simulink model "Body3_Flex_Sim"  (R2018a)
settings: Solver=ode3  StartTime=0.0  StopTime=200  FixedStep=Ts  RelTol=1e-3  EnableMultiTasking=on
InitFcn:
  | run
StopFcn:
  | pl
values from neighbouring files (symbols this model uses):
  d2r = pi/180    (= 0.0174532925199)    [orbitic.m]    (also in Quan.m; run.m; runf.m)
  Int_IC = [qti', 0 0, h0i(1:3)', 0 0, wr0, Vec0'*M0, Pec0']    [run.m]
  Kq1 = I22*ww^2 - 3*wo2*(I11-I33)    [run.m]
  Kq2 = 2*I22*zet*ww    [run.m]
  Kqi = 0.0005    [run.m]
  Kr1 = (0.1*I11*I33*zet^2/Hy0) - sqrt( ((0.01^zet^4*I11^2*I33^2)/Hy0^2)+(4*I11*I33*zet^2) )    [run.m]
  Kr2 = 0.05*Kr1    [run.m]
  Kr3 = 0.04*zet*(Kr2-Hy0) * sqrt(abs(Hy0/(I11*I33)))    [run.m]
  nt = 7    [run.m]    (also in runf.m)
  r2d = 180/pi    (= 57.2957795131)    [pl.m]    (also in pl2.m; run.m; plf.m; runf.m)
  Ts = 0.001    [run.m]    (also in runf.m = 0.0005)
  wo = 0.00113    [run.m]
undefined symbols (not defined in the file or in its folder): Aflx, Bflx, Cflx, den, Dflx, DiscIntNeverNeededParam, Mode_Switch, num, Phase_Plane, RW_Steering, Vehi_3B3W
libraries: simulink x4

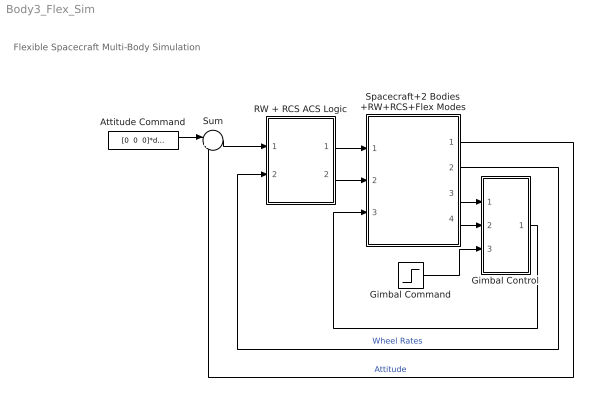
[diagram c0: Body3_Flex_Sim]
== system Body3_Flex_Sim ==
  note: Flexible Spacecraft Multi-Body Simulation
  Attitude Command : Constant  Value="[0  0  0]*d2r"
  Gimbal Control : Subsystem
  Gimbal Command : Step  After=[5, 5]*d2r  SampleTime=0
  RW + RCS ACS Logic : Subsystem
  Spacecraft+2 Bodies +RW+RCS+Flex Modes : Subsystem
  Sum : Sum  Inputs=|+-
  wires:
  Spacecraft+2 Bodies +RW+RCS+Flex Modes/2(Wrw) -> RW + RCS ACS Logic/2(wr(i))  "Wheel Rates"
  Attitude Command/1 -> Sum/1
  Spacecraft+2 Bodies +RW+RCS+Flex Modes/1(atti) -> Sum/2  "Attitude"
  Sum/1 -> RW + RCS ACS Logic/1(atter)
  RW + RCS ACS Logic/2(Trwi) -> Spacecraft+2 Bodies +RW+RCS+Flex Modes/2(Trw)
  RW + RCS ACS Logic/1(Frcs) -> Spacecraft+2 Bodies +RW+RCS+Flex Modes/1(Fjets)
  Spacecraft+2 Bodies +RW+RCS+Flex Modes/4(Gmb-dot) -> Gimbal Control/2(Grat)
  Spacecraft+2 Bodies +RW+RCS+Flex Modes/3(gimb) -> Gimbal Control/1(Gimb)
  Gimbal Control/1(Trq) -> Spacecraft+2 Bodies +RW+RCS+Flex Modes/3(Tgimb)
  Gimbal Command/1 -> Gimbal Control/3(Cmd)

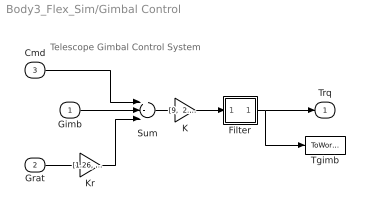
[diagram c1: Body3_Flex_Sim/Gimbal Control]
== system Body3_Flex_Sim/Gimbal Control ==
  note: Telescope Gimbal Control System
  Gimb : Inport
  Grat : Inport  Port=2
  Cmd : Inport  Port=3
  Filter : Subsystem
  K : Gain  Gain="[9,  2.85]"
  Kr : Gain  Gain="[1.26,  1.14]"
  Sum : Sum  Inputs=+--
  Tgimb : ToWorkspace  VariableName=Tgimb  SampleTime=-1
  Trq : Outport
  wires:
  K/1 -> Filter/1(I)
  Cmd/1 -> Sum/1
  Kr/1 -> Sum/3
  Grat/1 -> Kr/1
  Gimb/1 -> Sum/2
  Sum/1 -> K/1
  Filter/1(O) -> Tgimb/1, Trq/1

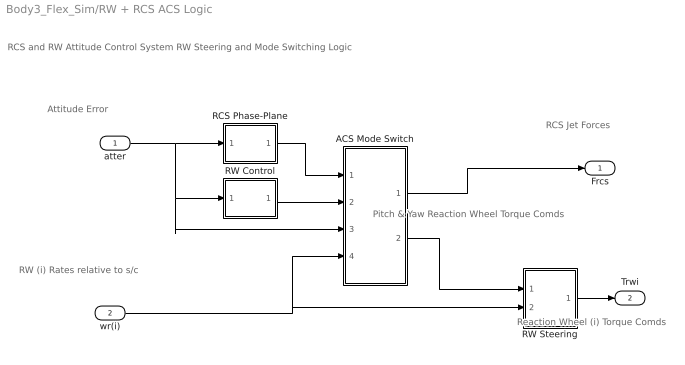
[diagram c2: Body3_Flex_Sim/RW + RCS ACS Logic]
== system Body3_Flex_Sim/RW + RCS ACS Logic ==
  note: RCS and RW Attitude Control System RW Steering and Mode Switching Logic
  note: RCS Jet Forces
  note: Reaction Wheel (i) Torque Comds
  note: RW (i) Rates relative to s/c
  note: Attitude Error
  note: Pitch & Yaw Reaction Wheel Torque Comds
  atter : Inport
  wr(i) : Inport  Port=2
  ACS Mode Switch : Subsystem
  RCS Phase-Plane : Subsystem
  RW Control : Subsystem
  RW Steering : Subsystem
  Frcs : Outport
  Trwi : Outport  Port=2
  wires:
  atter/1 -> ACS Mode Switch/3(atter), RW Control/1(atti), RCS Phase-Plane/1(atter)
  RW Control/1(Tc) -> ACS Mode Switch/2(Trw)
  RCS Phase-Plane/1(f(nt)) -> ACS Mode Switch/1(Frcs)
  ACS Mode Switch/2(" Trw") -> RW Steering/1(Trwc)
  wr(i)/1 -> RW Steering/2(wr(1)), ACS Mode Switch/4(wr(i))
  ACS Mode Switch/1(" Frcs") -> Frcs/1
  RW Steering/1(Twi) -> Trwi/1

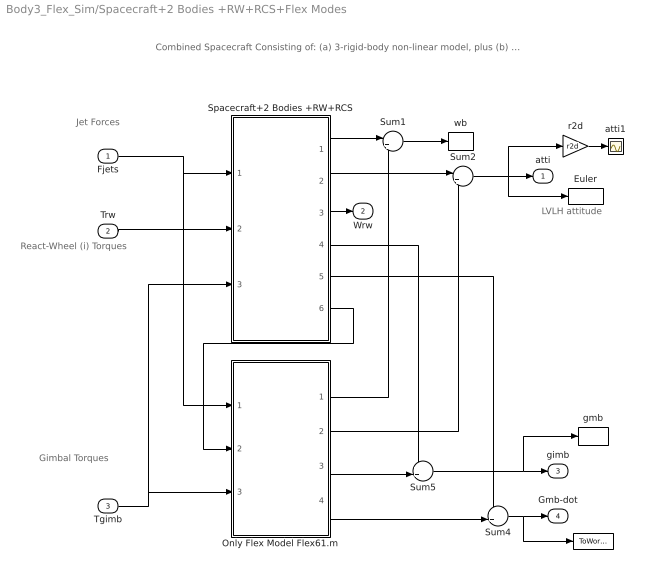
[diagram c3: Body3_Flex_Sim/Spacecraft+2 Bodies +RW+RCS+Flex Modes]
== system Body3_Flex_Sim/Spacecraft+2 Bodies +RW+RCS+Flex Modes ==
  note: LVLH attitude
  note: Combined Spacecraft Consisting of: (a) 3-rigid-body non-linear model, plus (b) a 61 flex modes state-space model
  note: Gimbal Torques
  note: Jet Forces
  note: React-Wheel (i) Torques
  Fjets : Inport
  Trw : Inport  Port=2
  Tgimb : Inport  Port=3
  "   " : ToWorkspace  VariableName=Gimdot  SampleTime=-1
  Euler : ToWorkspace  VariableName=Euler  SampleTime=-1
  Only Flex Model Flex61.m : Subsystem
  Spacecraft+2 Bodies +RW+RCS : Subsystem
  Sum1 : Sum  Inputs=|++
  Sum2 : Sum  Inputs=|++
  Sum4 : Sum  Inputs=++|
  Sum5 : Sum  Inputs=++|
  atti1 : Scope
  gmb : ToWorkspace  VariableName=Gimb  SampleTime=-1
  r2d : Gain  Gain=r2d
  wb : ToWorkspace  VariableName=wb  SampleTime=-1
  atti : Outport
  Wrw : Outport  Port=2
  gimb : Outport  Port=3
  Gmb-dot : Outport  Port=4
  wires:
  Fjets/1 -> Spacecraft+2 Bodies +RW+RCS/1(Frcs), Only Flex Model Flex61.m/1(Fjets)
  Trw/1 -> Spacecraft+2 Bodies +RW+RCS/2(Trw)
  Tgimb/1 -> Spacecraft+2 Bodies +RW+RCS/3(Tgimb), Only Flex Model Flex61.m/3(Tgimb)
  Spacecraft+2 Bodies +RW+RCS/1(W_b) -> Sum1/1
  Spacecraft+2 Bodies +RW+RCS/2(att) -> Sum2/1
  Spacecraft+2 Bodies +RW+RCS/4(gimb) -> Sum5/1
  Spacecraft+2 Bodies +RW+RCS/5(Gmb-dot) -> Sum4/1
  Spacecraft+2 Bodies +RW+RCS/3(Wrw) -> Wrw/1
  Sum1/1 -> wb/1
  Sum2/1 -> atti/1, Euler/1, r2d/1
  Sum5/1 -> gimb/1, gmb/1
  Sum4/1 -> Gmb-dot/1, "   "/1
  r2d/1 -> atti1/1
  Only Flex Model Flex61.m/2(atti) -> Sum2/2
  Only Flex Model Flex61.m/3(gimb) -> Sum5/2
  Only Flex Model Flex61.m/4(Gmb-dot) -> Sum4/2
  Only Flex Model Flex61.m/1(wb) -> Sum1/2
  Spacecraft+2 Bodies +RW+RCS/6(Twb) -> Only Flex Model Flex61.m/2(Trwb)

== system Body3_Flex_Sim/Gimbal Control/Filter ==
  I : Inport
  Demux : Demux  Outputs=2
  Filter1 : TransferFcn  Numerator=[80]  Denominator=[1 80]
  Filter2 : TransferFcn  Numerator=[80]  Denominator=[1 80]
  Mux : Mux  Inputs=2
  O : Outport
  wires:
  Mux/1 -> O/1
  I/1 -> Demux/1
  Demux/2 -> Filter2/1
  Demux/1 -> Filter1/1
  Filter2/1 -> Mux/2
  Filter1/1 -> Mux/1

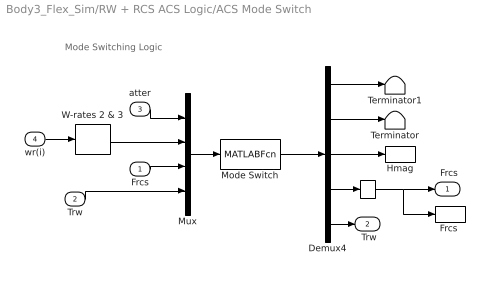
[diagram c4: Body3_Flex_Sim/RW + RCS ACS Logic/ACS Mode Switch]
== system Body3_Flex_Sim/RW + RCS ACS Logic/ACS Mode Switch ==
  note: Mode Switching Logic
  Frcs : Inport
  Trw : Inport  Port=2
  atter : Inport  Port=3
  wr(i) : Inport  Port=4
  "   " : Memory
  Demux4 : Demux  Outputs="[1 1 1 nt  2]"
  "Frcs " : ToWorkspace  VariableName=Frcs  SampleTime=-1
  Hmag : ToWorkspace  VariableName=Hmag  SampleTime=-1
  Mode Switch : MATLABFcn  MATLABFcn=Mode_Switch( u(1:3), u(4:5), u(6:5+nt), u(6+nt:7+nt) )  OutputDimensions=3+nt+2
  Mux : Mux  Inputs="[3  2  nt 2]"
  Terminator : Terminator
  Terminator1 : Terminator
  W-rates 2 & 3 : Selector  InputPortWidth=3  IndexOptions=Index vector (dialog)  Indices="[2  3]"  OutputSizes=1
  " Frcs" : Outport
  " Trw" : Outport  Port=2
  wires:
  Demux4/3 -> Hmag/1
  Demux4/2 -> Terminator/1
  Demux4/1 -> Terminator1/1
  W-rates 2 & 3/1 -> Mux/2
  "   "/1 -> "Frcs "/1, " Frcs"/1
  Demux4/5 -> " Trw"/1
  Demux4/4 -> "   "/1
  Mode Switch/1 -> Demux4/1
  Trw/1 -> Mux/4
  Frcs/1 -> Mux/3
  wr(i)/1 -> W-rates 2 & 3/1
  Mux/1 -> Mode Switch/1
  atter/1 -> Mux/1

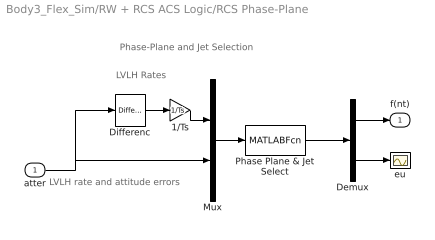
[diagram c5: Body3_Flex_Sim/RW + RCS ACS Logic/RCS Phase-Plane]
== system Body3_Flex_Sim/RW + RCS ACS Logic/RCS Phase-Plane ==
  note: Phase-Plane and Jet Selection
  note: LVLH Rates
  note: LVLH rate and attitude errors
  atter : Inport
  1/Ts : Gain  Gain=1/Ts
  Demux : Demux  Outputs=[nt, 3]
  Differenc : simulink/Discrete/Difference  ICPrevInput=0.0  InputProcessing=Inherited  OutMin=[]  OutMax=[]  OutDataType=sfix(16)  OutScaling=2^-10  DoSatur=off
  Mux : Mux  Inputs="[3  3]"
  Phase Plane & Jet Select : MATLABFcn  MATLABFcn=Phase_Plane( u(1:3), u(4:6) )  OutputDimensions=nt + 3
  eu : Scope
  f(nt) : Outport
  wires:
  Differenc/1 -> 1/Ts/1
  Mux/1 -> Phase Plane & Jet Select/1
  Phase Plane & Jet Select/1 -> Demux/1
  Demux/1 -> f(nt)/1
  Demux/2 -> eu/1
  1/Ts/1 -> Mux/1
  atter/1 -> Differenc/1, Mux/2

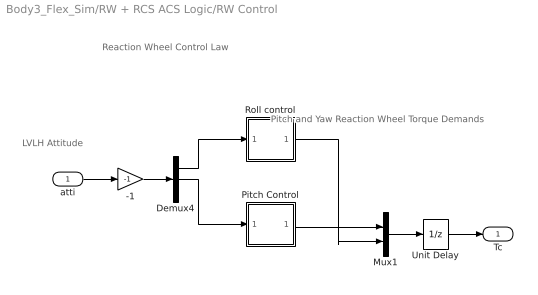
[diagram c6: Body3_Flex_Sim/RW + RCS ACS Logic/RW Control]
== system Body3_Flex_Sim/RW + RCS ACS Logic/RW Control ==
  note: Reaction Wheel Control Law
  note: LVLH Attitude
  note: Pitch and Yaw Reaction Wheel Torque Demands
  atti : Inport
  -1 : Gain  Gain=-1
  Demux4 : Demux  Outputs=3
  Mux1 : Mux  Inputs=2
  Pitch Control : Subsystem
  Roll control : Subsystem
  Unit Delay : UnitDelay  SampleTime=-1
  Tc : Outport
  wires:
  Unit Delay/1 -> Tc/1
  -1/1 -> Demux4/1
  Mux1/1 -> Unit Delay/1
  Roll control/1(Tcz) -> Mux1/2
  atti/1 -> -1/1
  Demux4/2 -> Pitch Control/1(the)
  Pitch Control/1(Tcy) -> Mux1/1
  Demux4/1 -> Roll control/1(phi)

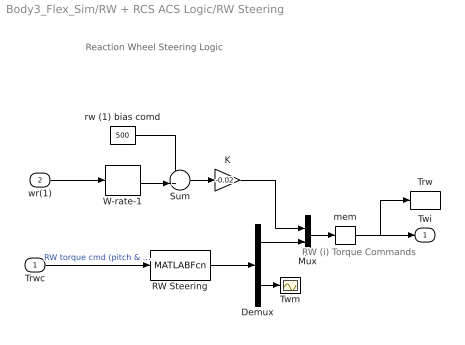
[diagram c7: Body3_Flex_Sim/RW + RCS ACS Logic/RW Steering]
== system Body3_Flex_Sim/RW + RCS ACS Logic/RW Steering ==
  note: RW (i) Torque Commands
  note: Reaction Wheel Steering Logic
  Trwc : Inport
  wr(1) : Inport  Port=2
  Demux : Demux  Outputs=[2, 1]
  K : Gain  Gain=-0.02
  Mux : Mux  Inputs=[1,2]
  RW Steering : MATLABFcn  MATLABFcn=RW_Steering( u(1:2) )  OutputDimensions=3
  Sum : Sum  Inputs=++|
  Trw : ToWorkspace  VariableName=Trw  SampleTime=-1
  Twm : Scope
  W-rate-1 : Selector  InputPortWidth=3  IndexOptions=Index vector (dialog)  Indices=[1]  OutputSizes=1
  mem : Memory
  rw (1) bias comd : Constant  Value=500
  Twi : Outport
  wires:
  Demux/2 -> Twm/1
  Demux/1 -> Mux/2
  RW Steering/1 -> Demux/1
  Trwc/1 -> RW Steering/1  "RW torque cmd (pitch & yaw)"
  Mux/1 -> mem/1
  wr(1)/1 -> W-rate-1/1
  Sum/1 -> K/1
  rw (1) bias comd/1 -> Sum/1
  W-rate-1/1 -> Sum/2
  K/1 -> Mux/1
  mem/1 -> Twi/1, Trw/1

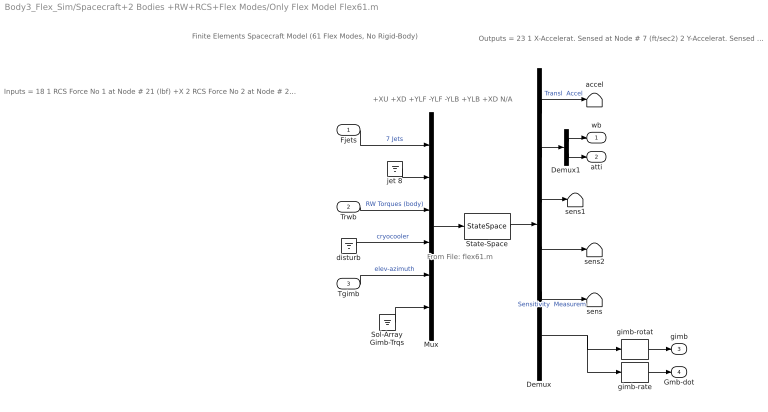
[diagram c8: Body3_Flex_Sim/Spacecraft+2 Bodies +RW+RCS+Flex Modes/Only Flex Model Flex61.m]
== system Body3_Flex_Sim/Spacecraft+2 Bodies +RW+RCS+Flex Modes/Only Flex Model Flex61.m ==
  note: From File: flex61.m
  note: +XU +XD +YLF -YLF -YLB +YLB +XD N/A
  note: Outputs = 23 1 X-Accelerat. Sensed at Node # 7 (ft/sec2) 2 Y-Accelerat. Sensed at Node # 7 (ft/sec2) 3 X-Rot. Rate Sensed at Node # 6 (radian) 4 Y-Rot. Rate Sensed at Node # 6 (radian) 5 Z-Rot. Rate Sensed at Node # 6 (radian) 6 X-Rotation Sensed at Node # 6 (radian) 7 Y-Rotation Sensed at Node # 6 (radian) 8 Z-Rotation Sensed at Node # 6 (radian) 9 Y-Rotation Mirror at Node # 9 (radian) 10 Z-Rotation Mirror at Node # 9 (radian) 11 Y-Rotation Instrum-2 Node # 10 (radian) 12 Z-Rotation Instrum-2 Node # 10 (radian) 13 X-Rotation Instrum-3 Node # 11 (radian) 14 Y-Rotation Instrum-4 Node # 12 (radian) 15 Z-Rotation Instrum-5 Node # 13 (radian) 16 Rotation Angle at Elevati Gimbal No 1 17 Rotation Rate at Elevati Gimbal No 1 18 Rotation Angle at Azimuth Gimbal No 2 19 Rotation Rate at Azimuth Gimbal No 2 20 Rotation Angle at Rght SA Gimbal No 3 21 Rotation Rate at Rght SA Gimbal No 3 22 Rotation Angle at Left SA Gimbal No 4 23 Rotation Rate at Left SA Gimbal No 4
  note: Inputs = 18 1 RCS Force No 1 at Node # 21 (lbf) +X 2 RCS Force No 2 at Node # 22 (lbf) +X 3 RCS Force No 3 at Node # 23 (lbf) +Y 4 RCS Force No 4 at Node # 24 (lbf) -Y 5 RCS Force No 5 at Node # 25 (lbf) -Y 6 RCS Force No 6 at Node # 26 (lbf) +Y 7 RCS Force No 7 at Node # 27 (lbf) +X 8 RCS Force No 8 at Node # 28 (lbf) +X 9 RW Torque No 1 at Node # 17 (ft-lb) roll 10 RW Torque No 2 at Node # 18 (ft-lb) ptch 11 RW Torque No 3 at Node # 19 (ft-lb) yaw 12 Dist Trque No 4 at Node # 8 (ft-lb) roll 13 Dist Trque No 5 at Node # 8 (ft-lb) ptch 14 Dist Trque No 6 at Node # 8 (ft-lb) yaw 15 Elevation Trqu at Gimbal No 1 (ft-lb) 16 Azimuth Torque at Gimbal No 2 (ft-lb) 17 Rght SA Torque at Gimbal No 3 (ft-lb) 18 Left SA Torque at Gimbal No 4 (ft-lb)
  note: Finite Elements Spacecraft Model (61 Flex Modes, No Rigid-Body)
  Fjets : Inport
  Trwb : Inport  Port=2
  Tgimb : Inport  Port=3
  Demux : Demux  Outputs="[2, 6, 2,2,3,  8]"
  Demux1 : Demux  Outputs=[3, 3]
  Mux : Mux  Inputs=[7,1,3,3,2,2]
  Sol-Array Gimb-Trqs : Ground
  State-Space : StateSpace  A=Aflx  B=Bflx  C=Cflx  D=Dflx  InitialCondition=0
  accel : Terminator
  disturb : Ground
  gimb-rate : Selector  InputPortWidth=8  IndexOptions=Index vector (dialog)  Indices=[2, 4]  OutputSizes=1
  gimb-rotat : Selector  InputPortWidth=8  IndexOptions=Index vector (dialog)  Indices=[1 3]  OutputSizes=1
  jet 8 : Ground
  sens : Terminator
  sens1 : Terminator
  sens2 : Terminator
  wb : Outport
  atti : Outport  Port=2
  gimb : Outport  Port=3
  Gmb-dot : Outport  Port=4
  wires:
  Demux1/2 -> atti/1
  Demux/5 -> sens/1  "Sensitivity  Measurem"
  Sol-Array Gimb-Trqs/1 -> Mux/6
  disturb/1 -> Mux/4  "cryocooler"
  Trwb/1 -> Mux/3  "RW Torques (body)"
  jet 8/1 -> Mux/2
  Fjets/1 -> Mux/1  "7 Jets"
  Mux/1 -> State-Space/1
  Demux1/1 -> wb/1
  Demux/2 -> Demux1/1
  State-Space/1 -> Demux/1
  Demux/1 -> accel/1  "Transl  Accel"
  Tgimb/1 -> Mux/5  "elev-azimuth"
  Demux/6 -> gimb-rate/1, gimb-rotat/1
  Demux/3 -> sens1/1
  Demux/4 -> sens2/1
  gimb-rate/1 -> Gmb-dot/1
  gimb-rotat/1 -> gimb/1

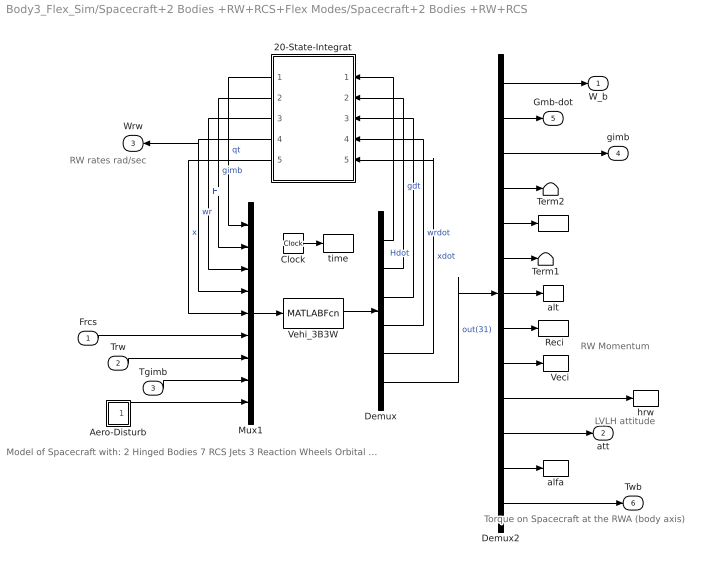
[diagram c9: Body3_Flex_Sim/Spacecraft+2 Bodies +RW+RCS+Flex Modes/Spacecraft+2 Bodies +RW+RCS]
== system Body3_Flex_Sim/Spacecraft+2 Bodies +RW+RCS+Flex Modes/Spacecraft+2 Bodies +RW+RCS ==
  note: RW Momentum
  note: Model of Spacecraft with: 2 Hinged Bodies 7 RCS Jets 3 Reaction Wheels Orbital Dynamics
  note: LVLH attitude
  note: Torque on Spacecraft at the RWA (body axis)
  note: RW rates rad/sec
  Frcs : Inport
  Trw : Inport  Port=2
  Tgimb : Inport  Port=3
  "    " : ToWorkspace  VariableName=hsys  SampleTime=-1
  "   Veci" : ToWorkspace  VariableName=Veci  SampleTime=-1
  "  Reci " : ToWorkspace  VariableName=Reci  SampleTime=-1
  20-State-Integrat : Subsystem
  Aero-Disturb : Subsystem
  Clock : Clock
  Demux : Demux  Outputs="[4,2,5,3,6,  31]"
  Demux2 : Demux  Outputs=[3,2,2,1, 3,2, 1,3,3,3,3, 2,3]
  Mux1 : Mux  Inputs="[4,2,5,3,6,  nt,3,2,3]"
  Term1 : Terminator
  Term2 : Terminator
  Vehi_3B3W : MATLABFcn  MATLABFcn=Vehi_3B3W( u(1:20), u(21:20+nt), u(21+nt:23+nt), u(24+nt:25+nt), u(26+nt:28+nt) )  OutputDimensions=51
  alfa : ToWorkspace  VariableName=alfa  SampleTime=-1
  alt : ToWorkspace  VariableName=alt  SampleTime=-1
  hrw : ToWorkspace  VariableName=hrw  SampleTime=-1
  time : ToWorkspace  VariableName=time  SampleTime=-1
  W_b : Outport
  att : Outport  Port=2
  Wrw : Outport  Port=3
  gimb : Outport  Port=4
  Gmb-dot : Outport  Port=5
  Twb : Outport  Port=6
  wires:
  Demux2/9 -> "   Veci"/1
  Vehi_3B3W/1 -> Demux/1
  20-State-Integrat/1(qt) -> Mux1/1  "qt"
  20-State-Integrat/2(gimb) -> Mux1/2  "gimb"
  20-State-Integrat/3(H) -> Mux1/3  "H"
  20-State-Integrat/4(wr) -> Wrw/1, Mux1/4  "wr"
  20-State-Integrat/5(x) -> Mux1/5  "x"
  Demux/6 -> Demux2/1  "out(31)"
  Demux/1 -> 20-State-Integrat/1(qdot)
  Demux/2 -> 20-State-Integrat/2(gmbdot)  "gdt"
  Demux/3 -> 20-State-Integrat/3(Hdot)  "Hdot"
  Demux/4 -> 20-State-Integrat/4(wrdor)  "wrdot"
  Demux/5 -> 20-State-Integrat/5(xdot)  "xdot"
  Demux2/12 -> alfa/1
  Demux2/11 -> att/1
  Demux2/10 -> hrw/1
  Demux2/8 -> "  Reci "/1
  Demux2/7 -> alt/1
  Demux2/5 -> "    "/1
  Demux2/6 -> Term1/1
  Demux2/1 -> W_b/1
  Demux2/4 -> Term2/1
  Demux2/2 -> Gmb-dot/1
  Demux2/3 -> gimb/1
  Clock/1 -> time/1
  Tgimb/1 -> Mux1/8
  Trw/1 -> Mux1/7
  Mux1/1 -> Vehi_3B3W/1
  Demux2/13 -> Twb/1
  Frcs/1 -> Mux1/6
  Aero-Disturb/1(Td) -> Mux1/9

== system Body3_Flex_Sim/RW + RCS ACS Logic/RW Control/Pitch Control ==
  note: Pitch Control Logic
  the : Inport
  Differenc : simulink/Discrete/Difference  ICPrevInput=-0.1757  InputProcessing=Inherited  OutMin=[]  OutMax=[]  OutDataType=sfix(16)  OutScaling=2^-10  DoSatur=off
  Integrator : DiscreteIntegrator  SampleTime=Ts  ICPrevOutput=DiscIntNeverNeededParam  ICPrevScaledInput=DiscIntNeverNeededParam
  Kq1 : Gain  Gain=Kq1
  Kq2/Ts : Gain  Gain=Kq2/Ts
  Kqi : Gain  Gain=Kqi
  Sum4 : Sum  Inputs=+++
  Tcy : Outport
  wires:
  Kq2/Ts/1 -> Sum4/1
  Differenc/1 -> Kq2/Ts/1
  Integrator/1 -> Kqi/1
  Kqi/1 -> Sum4/3
  the/1 -> Integrator/1, Differenc/1, Kq1/1
  Sum4/1 -> Tcy/1
  Kq1/1 -> Sum4/2

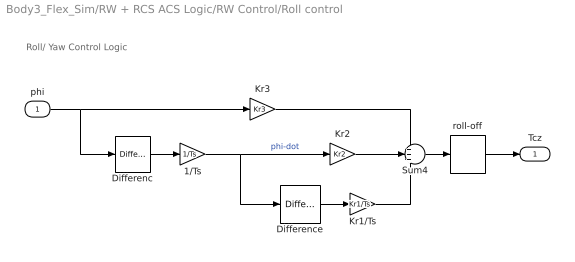
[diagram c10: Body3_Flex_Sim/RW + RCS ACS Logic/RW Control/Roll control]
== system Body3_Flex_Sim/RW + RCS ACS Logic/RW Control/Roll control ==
  note: Roll/ Yaw Control Logic
  phi : Inport
  1/Ts : Gain  Gain=1/Ts
  Differenc : simulink/Discrete/Difference  ICPrevInput=0  InputProcessing=Inherited  OutMin=[]  OutMax=[]  OutDataType=sfix(16)  OutScaling=2^-10  DoSatur=off
  Difference : simulink/Discrete/Difference  ICPrevInput=0.0  InputProcessing=Inherited  OutMin=[]  OutMax=[]  OutDataType=sfix(16)  OutScaling=2^-10  DoSatur=off
  Kr1/Ts : Gain  Gain=Kr1/Ts
  Kr2 : Gain  Gain=Kr2
  Kr3 : Gain  Gain=Kr3
  Sum4 : Sum  Inputs=+++
  roll-off : DiscreteTransferFcn  Numerator=[num]  Denominator=[den]  SampleTime=Ts
  Tcz : Outport
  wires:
  roll-off/1 -> Tcz/1
  1/Ts/1 -> Difference/1, Kr2/1  "phi-dot"
  Differenc/1 -> 1/Ts/1
  Difference/1 -> Kr1/Ts/1
  Sum4/1 -> roll-off/1
  phi/1 -> Differenc/1, Kr3/1
  Kr1/Ts/1 -> Sum4/3
  Kr2/1 -> Sum4/2
  Kr3/1 -> Sum4/1

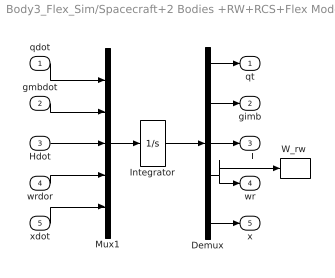
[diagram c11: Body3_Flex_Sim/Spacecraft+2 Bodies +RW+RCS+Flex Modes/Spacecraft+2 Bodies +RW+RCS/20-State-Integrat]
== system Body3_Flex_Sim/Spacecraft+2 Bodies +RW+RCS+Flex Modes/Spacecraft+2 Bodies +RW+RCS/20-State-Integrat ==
  qdot : Inport
  gmbdot : Inport  Port=2
  Hdot : Inport  Port=3
  wrdor : Inport  Port=4
  xdot : Inport  Port=5
  Demux : Demux  Outputs=[4,2,5,3,6]
  Integrator : Integrator  InitialCondition=Int_IC
  Mux1 : Mux  Inputs=[4,2,5,3,6]
  "W_rw " : ToWorkspace  VariableName=W_rw  SampleTime=-1
  qt : Outport
  gimb : Outport  Port=2
  H : Outport  Port=3
  wr : Outport  Port=4
  x : Outport  Port=5
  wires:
  Demux/5 -> x/1
  Demux/4 -> wr/1, "W_rw "/1
  Demux/3 -> H/1
  Demux/2 -> gimb/1
  Demux/1 -> qt/1
  xdot/1 -> Mux1/5
  wrdor/1 -> Mux1/4
  Hdot/1 -> Mux1/3
  gmbdot/1 -> Mux1/2
  qdot/1 -> Mux1/1
  Integrator/1 -> Demux/1
  Mux1/1 -> Integrator/1

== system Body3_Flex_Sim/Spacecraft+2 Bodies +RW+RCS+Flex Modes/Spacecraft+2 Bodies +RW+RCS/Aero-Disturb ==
  note: Aerodynamic Disturbance Torques
  30 : Gain  Gain=30
  Disturb Trq1 : Sin  Amplitude="[0.0,   1,   0.2]*0.0001"  Bias="[0.0,  0.5,  0.15]*0.0001"  Frequency=[wo, wo, wo]  SampleTime=0
  Disturb Trq2 : Sin  Amplitude=[0, 1.2, 1]*0.0001  Bias=[0 0 0]  Frequency=[wo, wo, wo]*2  SampleTime=0
  Sum2 : Sum  Inputs=+|+
  "Td " : ToWorkspace  VariableName=Td  SampleTime=-1
  Td : Outport
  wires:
  30/1 -> "Td "/1, Td/1
  Disturb Trq2/1 -> Sum2/2  "2*wo"
  Sum2/1 -> 30/1
  Disturb Trq1/1 -> Sum2/1  "wo"
